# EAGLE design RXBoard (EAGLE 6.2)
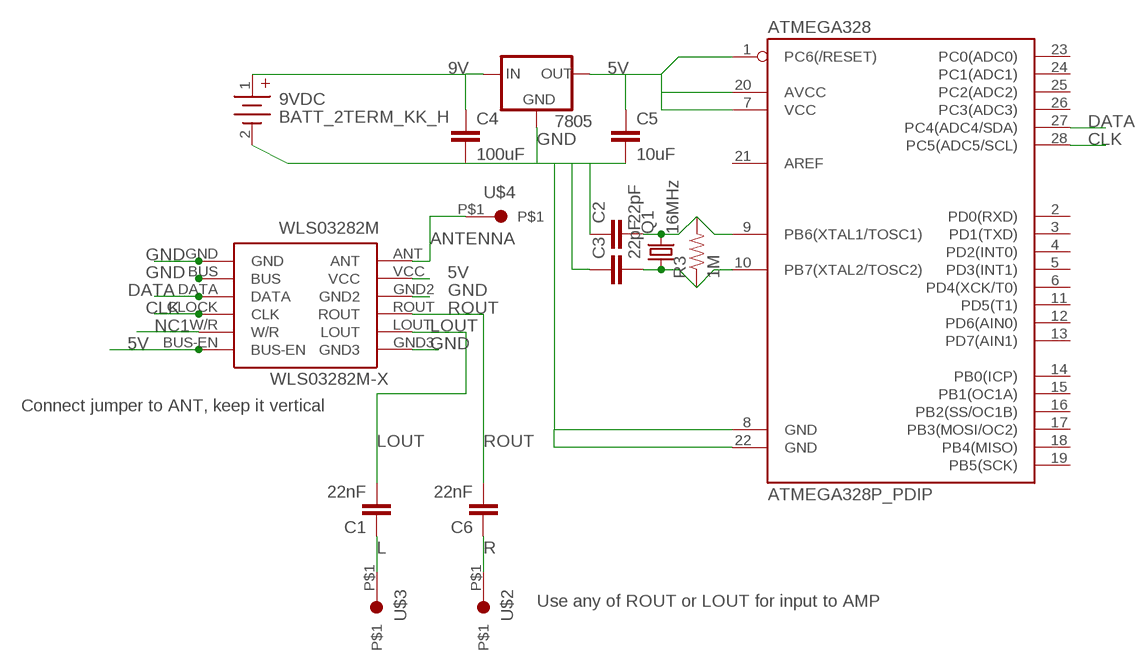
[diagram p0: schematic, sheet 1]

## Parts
9VDC  BATT_2TERM_KK_H  [KK-H-2]
7805  V_REG_78XXSIDE  [78XXL]
ATMEGA328  ATMEGA328P_PDIP  [DIL28-3]
C1  22nF  CAPPTH  [CAP-PTH-SMALL]
C2  22pF  CAPPTH  [CAP-PTH-SMALL]
C3  22pF  CAPPTH  [CAP-PTH-SMALL]
C4  100uF  CAPPTH  [CAP-PTH-SMALL]
C5  10uF  CAPPTH  [CAP-PTH-SMALL]
C6  22nF  CAPPTH  [CAP-PTH-SMALL]
Q1  16MHz  CRYSTALHC18U-V  [HC18U-V]
R3  1M  RESISTORAXIAL-0.3  [AXIAL-0.3]
U$2  JUMPERDOT  [JUMPERDOT]
U$3  JUMPERDOT  [JUMPERDOT]
U$4  JUMPERDOT  [JUMPERDOT]
WLS03282M  WLS03282M-X  [WLS..PCB]

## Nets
5V: 7805.OUT ATMEGA328.1(PC6(/RESET)) ATMEGA328.7(VCC) ATMEGA328.20(AVCC) C5.1 WLS03282M.BUS-EN WLS03282M.VCC
9V: 9VDC.1 7805.IN C4.1
ANTENNA: U$4.P$1 WLS03282M.ANT
CLK: ATMEGA328.28(PC5(ADC5/SCL)) WLS03282M.CLOCK(CLK)
DATA: ATMEGA328.27(PC4(ADC4/SDA)) WLS03282M.DATA
GND: 9VDC.2 7805.GND ATMEGA328.8(GND) ATMEGA328.22(GND) C2.1 C3.1 C4.2 C5.2 WLS03282M.BUS WLS03282M.GND WLS03282M.GND2 WLS03282M.GND3
L: C1.1 U$3.P$1
LOUT: C1.2 WLS03282M.LOUT
N$1: ATMEGA328.9(PB6(XTAL1/TOSC1)) C2.2 Q1.2 R3.P$2
N$2: ATMEGA328.10(PB7(XTAL2/TOSC2)) C3.2 Q1.1 R3.P$1
NC1: WLS03282M.W/R
R: C6.1 U$2.P$1
ROUT: C6.2 WLS03282M.ROUT
Unconnected: ATMEGA328.2(PD0(RXD)) ATMEGA328.3(PD1(TXD)) ATMEGA328.4(PD2(INT0)) ATMEGA328.5(PD3(INT1)) ATMEGA328.6(PD4(XCK/T0)) ATMEGA328.11(PD5(T1)) ATMEGA328.12(PD6(AIN0)) ATMEGA328.13(PD7(AIN1)) ATMEGA328.14(PB0(ICP)) ATMEGA328.15(PB1(OC1A)) ATMEGA328.16(PB2(SS/OC1B)) ATMEGA328.17(PB3(MOSI/OC2)) ATMEGA328.18(PB4(MISO)) ATMEGA328.19(PB5(SCK)) ATMEGA328.21(AREF) ATMEGA328.23(PC0(ADC0)) ATMEGA328.24(PC1(ADC1)) ATMEGA328.25(PC2(ADC2)) ATMEGA328.26(PC3(ADC3))

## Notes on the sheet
- Connect jumper to ANT, keep it vertical
- Use any of ROUT or LOUT for input to AMP

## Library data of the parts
9VDC = battery:BATT_2TERM_*: Molex KK
7805 = SparkFun-PowerIC:V_REG_78XX: Voltage Regulator Standard 7805 5V regulator. IGO (Input Ground Output). Spark Fun Electronics SKU : COM-00107
ATMEGA328 = SparkFun-DigitalIC:ATMEGA328P_PDIP: uC used in the Arduino 32kb flash, 1k EEPROM, 2k SRAM This is the through-hole version of this chip.
C1-C6 = SparkFun-Passives:CAP: Capacitor
Q1 = crystal:CRYSTAL: CRYSTAL; OC_FARNELL: unknown; OC_NEWARK: unknown
R3 = SparkFun-Passives:RESISTOR: Resistor
U$2-U$4 = fz:JUMPERDOT
WLS03282M = fz:WLS03282M

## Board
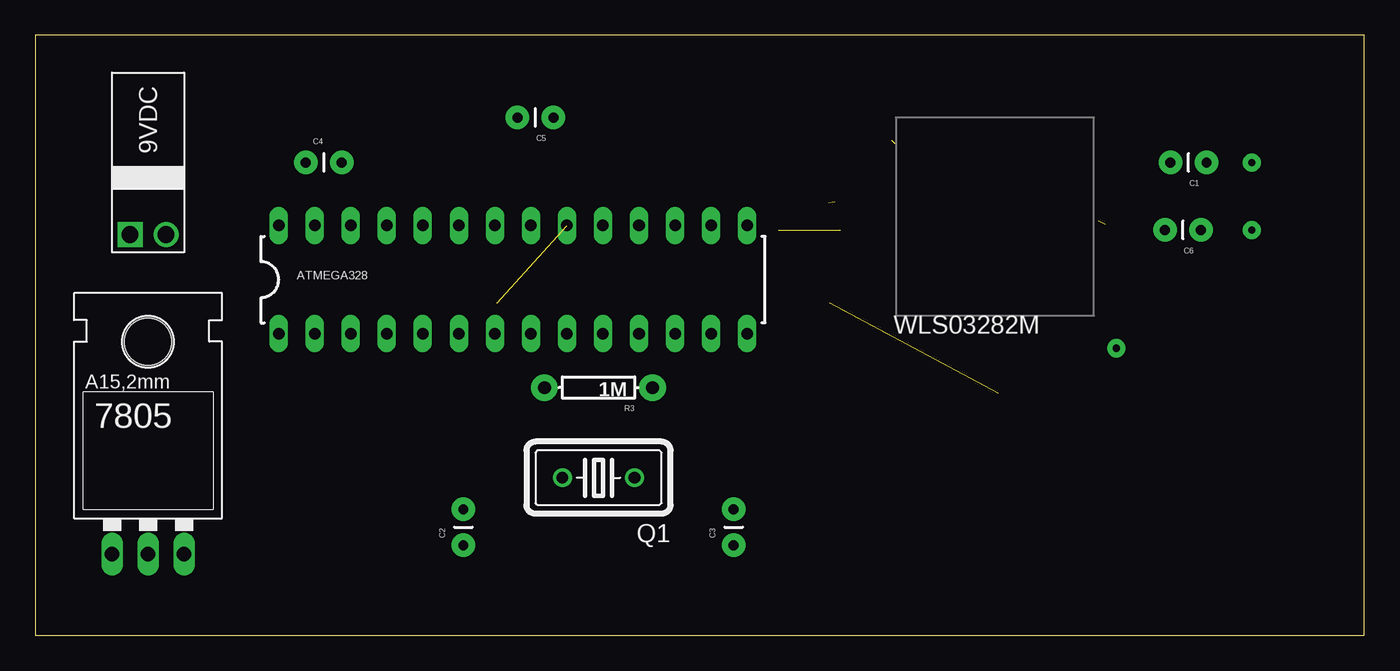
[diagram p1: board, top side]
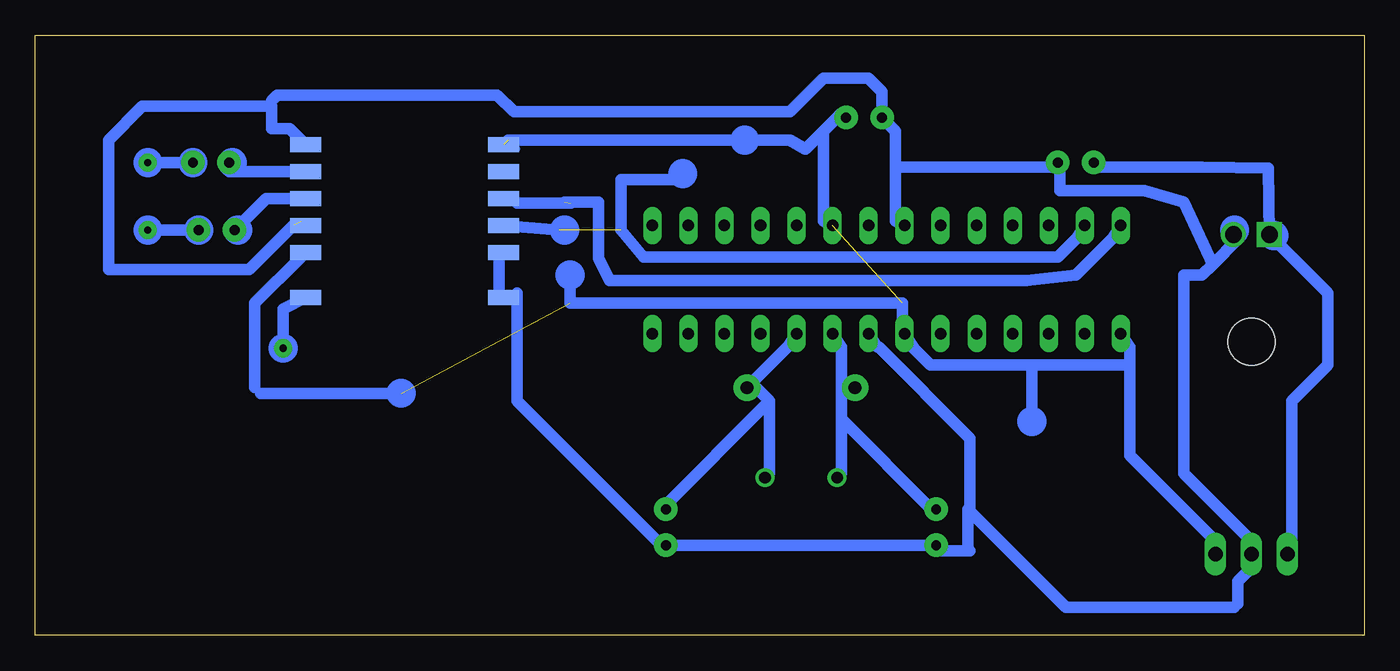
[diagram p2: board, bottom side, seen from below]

Size 93.65 x 42.3 mm. Coordinates in mm from the lower left corner, seen from the top.
Outline: 0,0 93.65,0 93.65,42.3 0,42.3 0,0
Copper layers (1*16): Top 0.035mm / dielectric 1.5mm / Bottom 0.035mm
Design rules: minimum track width 10mil, minimum drill 24mil, track to track 8mil, track to pad 8mil, pad to pad 8mil, via to via 8mil, smd to smd 8mil, copper to edge 40mil, drill to drill 8mil, minimum pad ring 10mil, minimum via ring 8mil, stop-mask expansion 4mil, vias tented up to drill 0mil, thermal gap 10mil

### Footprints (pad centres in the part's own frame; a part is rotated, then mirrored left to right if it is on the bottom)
KK-H-2 = drill 1.168 square: 1 -5.08,1.27 | drill 1.168: 2 -5.08,-1.27
78XXL = drill 1.016 long: GND 0,-3.81; IN -2.54,-3.81; OUT 2.54,-3.81 | hole 3.302: 0,11.176
DIL28-3 = drill 0.813 long: 1 -16.51,-3.81; 2 -13.97,-3.81; 3 -11.43,-3.81; 4 -8.89,-3.81; 5 -6.35,-3.81; 6 -3.81,-3.81; 7 -1.27,-3.81; 8 1.27,-3.81; 9 3.81,-3.81; 10 6.35,-3.81; 11 8.89,-3.81; 12 11.43,-3.81; 13 13.97,-3.81; 14 16.51,-3.81; 15 16.51,3.81; 16 13.97,3.81; 17 11.43,3.81; 18 8.89,3.81; 19 6.35,3.81; 20 3.81,3.81; 21 1.27,3.81; 22 -1.27,3.81; 23 -3.81,3.81; 24 -6.35,3.81; 25 -8.89,3.81; 26 -11.43,3.81; 27 -13.97,3.81; 28 -16.51,3.81
CAP-PTH-SMALL = drill 0.7 pad 1.651: 1 0,0; 2 2.54,0
HC18U-V = drill 0.813: 1 -2.54,0; 2 2.54,0
AXIAL-0.3 = drill 0.9 pad 1.88: P$1 -3.81,0; P$2 3.81,0
JUMPERDOT = drill 0.5 pad 1.27: P$1 0,0
WLS..PCB = smd 2.184 x 1.067 bottom: ANT 0,12.7; BUS 13.97,9.525; BUS-EN 13.97,1.905; CLOCK 13.97,5.715; DATA 13.97,7.62; GND 13.97,12.7; GND2 0,7.62; GND3 0,1.905; LOUT 0,3.81; ROUT 0,5.715; VCC 0,9.525; W/R 13.97,3.81

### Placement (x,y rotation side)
9VDC  7.94,33.34 90 top
7805  7.94,9.53 0 top
ATMEGA328  33.66,25.08 0 top
C1  82.55,33.34 180 top
C2  30.16,6.35 90 top
C3  49.21,6.35 90 top
C4  19.05,33.34 0 top
C5  36.51,36.51 180 top
C6  82.15,28.57 180 top
Q1  39.69,11.11 180 top
R3  39.69,17.46 180 top
U$2  85.72,28.57 0 top
U$3  85.72,33.34 0 top
U$4  76.2,20.24 0 top
WLS03282M  74.61,36.51 180 top

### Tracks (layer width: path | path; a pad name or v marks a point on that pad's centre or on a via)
5V  (3 unrouted)
  Bottom 0.254: 74.93,26.67 WLS03282M.VCC
  Bottom 0.406: 31.75,20.32 30.48,19.05 30.56,19.05 | 59.69,34.29 WLS03282M.BUS-EN 60.96,34.29 | 78.18,17.46 77.79,17.07
  Bottom 0.813: 16.51,19.05 16.51,12.7 10.16,6.35 7805.OUT | 16.51,19.05 16.51,20.32 ATMEGA328.1 | 16.51,19.05 23.42,19.05 | 23.42,19.05 30.48,19.05 | 31.75,20.32 ATMEGA328.7 | 38.1,35.56 36.83,36.83 C5.1 | 38.1,35.56 39.37,34.29 40.48,34.92 60.33,34.92 | 38.1,35.56 38.1,29.21 ATMEGA328.20 | 74.93,26.67 78.18,23.42 78.18,17.46 | 77.79,17.07 67.87,17.07 | 30.56,19.05 32.54,21.03 32.54,23.42 55.96,23.42 55.96,25.4 | 23.42,19.05 23.42,15.08
9V
  Bottom 0.406: 5.08,6.35 7805.IN | 19.05,33.02 C4.1
  Bottom 0.813: 5.08,6.35 5.08,16.51 2.54,19.05 2.54,24.13 9VDC.1 6.75,32.94 11.43,33.02 19.05,33.02
ANTENNA
  Bottom 0.813: WLS03282M.ANT 76.2,23.02 U$4.P$1
CLK  (1 unrouted)
  Bottom 0.254: 59.69,30.48 WLS03282M.CLOCK
  Bottom 0.813: 55.88,30.48 59.69,30.48 | ATMEGA328.28 17.78,27.94 20.32,25.4 23.81,25 53.18,25 53.98,26.59 53.98,30.56 56.36,30.56
DATA  (1 unrouted)
  Bottom 0.254: 60.96,29.21 WLS03282M.DATA
  Bottom 0.406: 52.39,28.57 52.39,30.96
  Bottom 0.813: ATMEGA328.27 20.32,27.94 21.59,26.67 50.8,26.67 52.39,28.57 | WLS03282M.DATA 56.75,28.57
GND  (1 unrouted)
  Bottom 0.254: 59.69,24.13 WLS03282M.GND | 30.48,6.35 C2.1
  Bottom 0.406: 74.93,29.21 WLS03282M.GND2 | WLS03282M.GND3 74.93,34.29 74.93,34.85 75.8,35.72 75.72,35.72 | 60.96,24.13 WLS03282M.GND | 60.96,26.67 WLS03282M.BUS | 49.53,6.35 C3.1 | 21.59,33.02 C4.2 21.43,33.18 | 34.29,20.32 34.21,20.32 | 27.78,9.05 27.94,8.89 | 27.94,6.11 27.78,5.95 | 29.77,5.95 C2.1 | 8.89,2.22 9.13,1.98 | 76.99,37.7 76.99,37.31
  Bottom 0.813: 33.02,33.02 33.02,35.56 C5.2 33.97,38.34 34.92,39.29 38.1,39.29 40.48,36.91 59.93,36.91 61.12,38.1 76.6,38.1 76.99,37.7 | 33.02,33.02 33.02,29.21 ATMEGA328.22 | 33.02,33.02 21.59,33.02 | 60.96,26.67 60.96,24.13 | 59.69,24.13 59.69,16.51 49.53,6.35 | 34.29,20.32 ATMEGA328.8 | 10.68,26.15 11.43,25.4 12.7,25.4 12.7,11.43 7.62,6.35 7805.GND 7.62,5.08 8.89,3.81 8.89,2.22 | 10.68,26.15 8.89,27.94 9VDC.2 | 30.48,6.35 C3.1 | 34.21,20.32 27.78,13.89 27.78,9.05 | 27.94,6.11 27.94,8.89 21.03,1.98 9.13,1.98 | 27.78,5.95 29.77,5.95 | 21.43,33.18 21.43,31.35 15.48,31.35 12.7,30.56 10.68,26.15 | 75.72,35.72 WLS03282M.GND3 | 75.8,35.72 76.99,35.72 76.99,37.31 86.12,37.31 88.5,34.92 88.5,25.8 78.58,25.8 75.41,28.97
L
  Bottom 0.813: C1.1 U$3.P$1
LOUT
  Bottom 0.254: 73.66,33.02 WLS03282M.LOUT
  Bottom 0.406: 80.01,32.7 C1.2
  Bottom 0.813: WLS03282M.LOUT 80.01,32.7
N$1
  Bottom 0.813: 36.83,17.78 36.83,20.32 ATMEGA328.9 | 36.83,17.78 36.83,15.24 | 36.83,15.24 36.83,11.43 Q1.2 | 36.83,15.24 30.48,8.89 C2.2 | 36.83,17.78 35.56,17.78 R3.P$2
N$2
  Bottom 0.254: 49.53,8.89 C3.2
  Bottom 0.406: 43.18,17.78 R3.P$1
  Bottom 0.813: 41.91,16.51 41.91,11.43 Q1.1 | 41.91,16.51 43.18,17.78 40.64,20.32 ATMEGA328.10 | 41.91,16.51 49.53,8.89
N$4
  Bottom 0.813: 48.02,32.15 52.39,32.15 52.39,28.57
R
  Bottom 0.813: C6.1 U$2.P$1
ROUT
  Bottom 0.254: 73.66,30.48 WLS03282M.ROUT
  Bottom 0.813: WLS03282M.ROUT 77.39,30.8 C6.2
(copper drawn outside any net)
  shapes: Bottom circle x15

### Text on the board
tDocu: Ajmp | Bjmp | Bjmp | Cjmp | Cjmp | Ajmp

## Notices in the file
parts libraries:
SparkFun-DigitalIC: Licensing: CC v3.0 Share-Alike You are welcome to use this library for commercial purposes.
